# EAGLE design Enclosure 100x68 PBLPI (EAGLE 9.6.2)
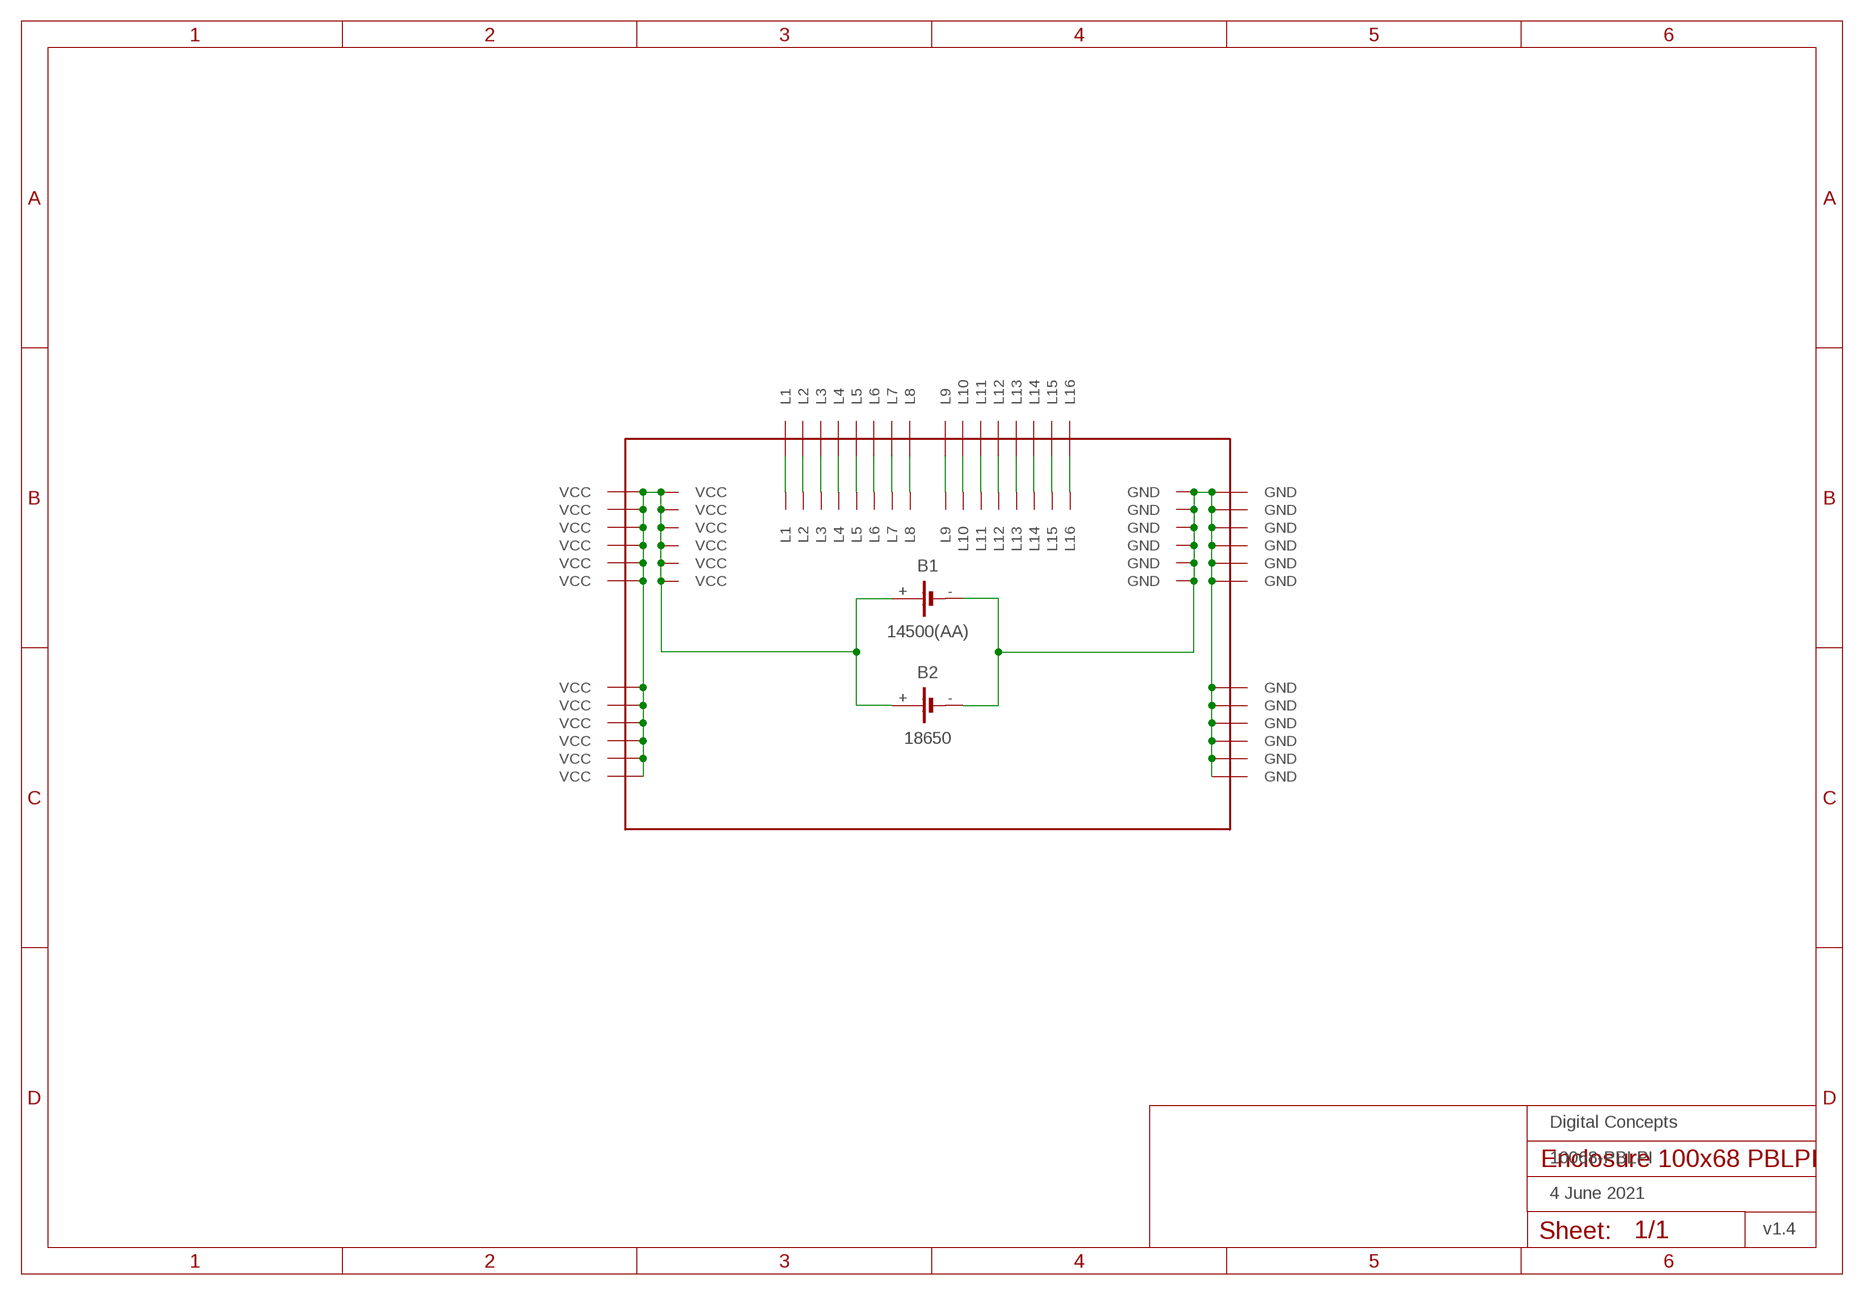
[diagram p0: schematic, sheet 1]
FRAME1 (FRAME-A4L-LOC): DATE: 4 June 2021; OWNER: Digital Concepts; TITLE: 10068-PBLPI; VERSION: v1.4

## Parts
B1  14500(AA)  BATTERY-HOLDER-14500(AA)  [BATTERY-14500]
B2  18650  BATTERY-HOLDER-18650  [BATTERY-18650]
P1  PROTO-34X22-BAT-PI  [PROTO-34X22-BAT-PI]

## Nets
GND: B1.- B2.- P1.P33-13(GND) P1.P33-14(GND) P1.P33-15(GND) P1.P33-16(GND) P1.P33-17(GND) P1.P33-18(GND) P1.P34-05(GND) P1.P34-06(GND) P1.P34-07(GND) P1.P34-08(GND) P1.P34-09(GND) P1.P34-10(GND) P1.P34-13(GND) P1.P34-14(GND) P1.P34-15(GND) P1.P34-16(GND) P1.P34-17(GND) P1.P34-18(GND)
N$1: P1.P10-21(L1) P1.P10-22(L1)
N$2: P1.P11-21(L2) P1.P11-22(L2)
N$3: P1.P12-21(L3) P1.P12-22(L3)
N$4: P1.P13-21(L4) P1.P13-22(L4)
N$5: P1.P14-21(L5) P1.P14-22(L5)
N$6: P1.P15-21(L6) P1.P15-22(L6)
N$7: P1.P16-21(L7) P1.P16-22(L7)
N$8: P1.P17-21(L8) P1.P17-22(L8)
N$9: P1.P18-21(L9) P1.P18-22(L9)
N$10: P1.P19-21(L10) P1.P19-22(L10)
N$11: P1.P20-21(L11) P1.P20-22(L11)
N$12: P1.P21-21(L12) P1.P21-22(L12)
N$13: P1.P22-21(L13) P1.P22-22(L13)
N$14: P1.P23-21(L14) P1.P23-22(L14)
N$15: P1.P24-21(L15) P1.P24-22(L15)
N$16: P1.P25-21(L16) P1.P25-22(L16)
VCC: B1.+ B2.+ P1.P01-05(VCC) P1.P01-06(VCC) P1.P01-07(VCC) P1.P01-08(VCC) P1.P01-09(VCC) P1.P01-10(VCC) P1.P01-13(VCC) P1.P01-14(VCC) P1.P01-15(VCC) P1.P01-16(VCC) P1.P01-17(VCC) P1.P01-18(VCC) P1.P02-13(VCC) P1.P02-14(VCC) P1.P02-15(VCC) P1.P02-16(VCC) P1.P02-17(VCC) P1.P02-18(VCC)

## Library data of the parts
B1 = digitalconcepts:BATTERY-HOLDER-14500(AA): 14500 (AA) battery holder
B2 = digitalconcepts:BATTERY-HOLDER-18650: 18650 Battery Holder
P1 = digitalconcepts:PROTO-34X22-BAT-PI: 34 x 22 Prototyping board, with battery connection (GND + Vcc plane), coupled side connection and Raspberry Pi Zero standoff mounting points, to fit a 100 x 68 enclosure

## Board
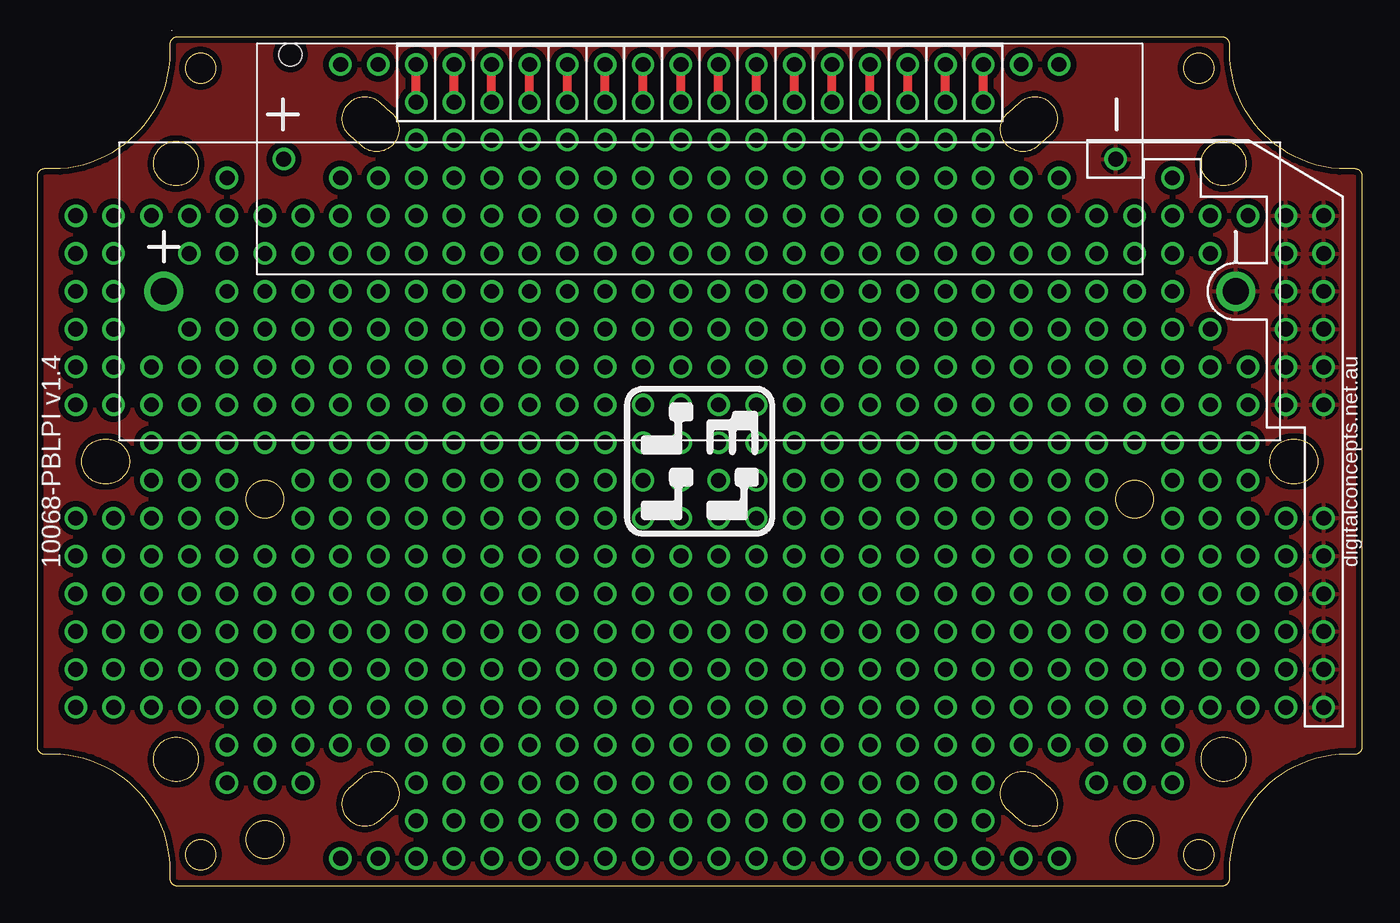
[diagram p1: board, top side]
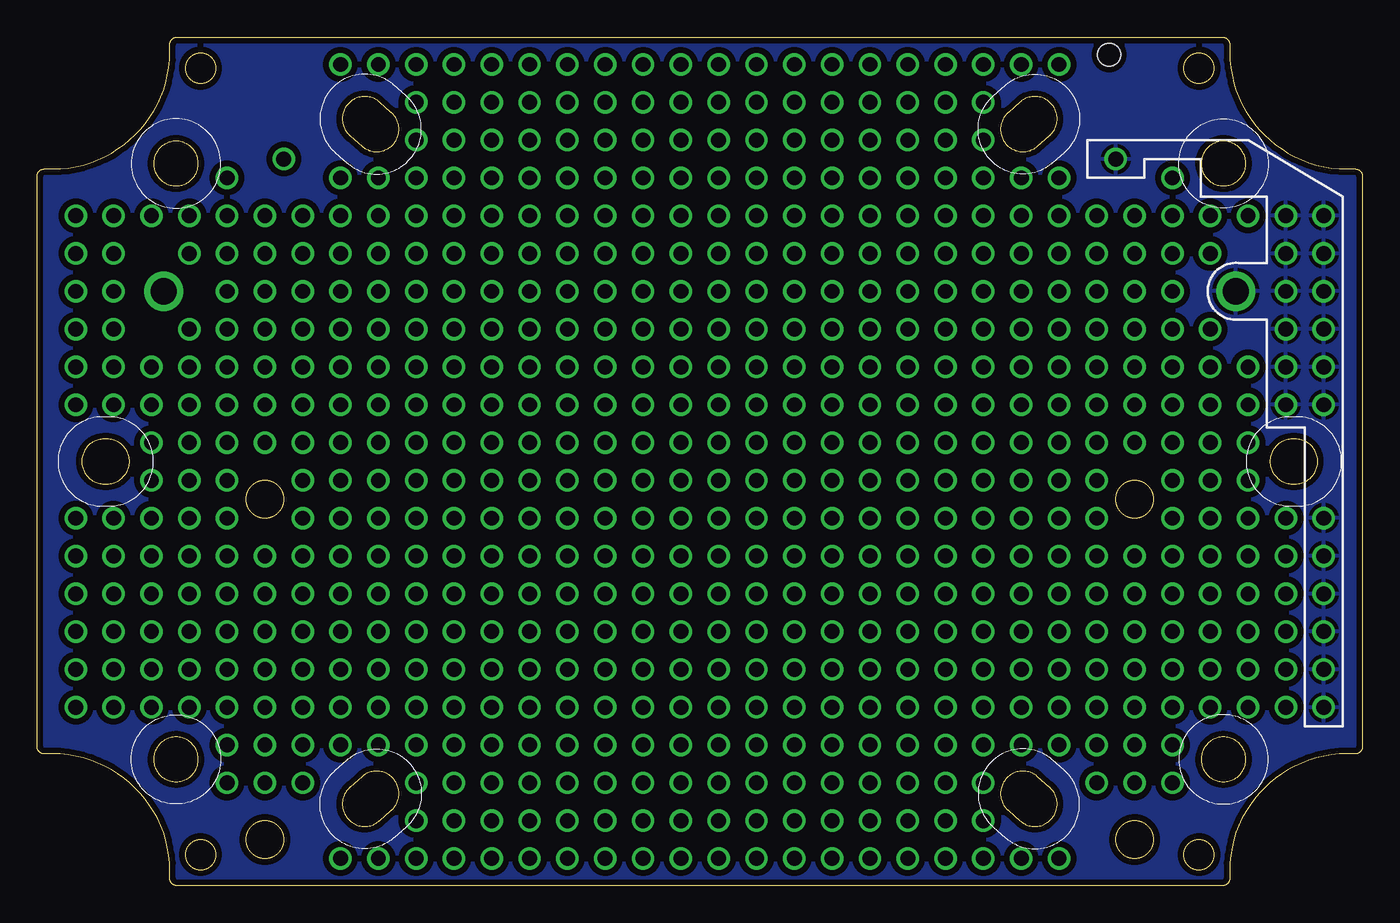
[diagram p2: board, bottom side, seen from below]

Size 89 x 57 mm. Coordinates in mm from the lower left corner, seen from the top.
Outline: 1238 segments
Outline: circle at 15.29,25.96 radius 1.27
Outline: circle at 15.29,3.1 radius 1.27
Outline: circle at 73.71,3.1 radius 1.27
Outline: circle at 73.71,25.96 radius 1.27
Outline: circle at 10.97,54.92 radius 1.02
Outline: circle at 10.97,2.08 radius 1.02
Outline: circle at 78.03,2.08 radius 1.02
Outline: circle at 78.03,54.92 radius 1.02
Copper layers (1*16): Top 0.035mm / dielectric 1.5mm / Bottom 0.035mm
Design rules "default *": minimum track width 6mil, minimum drill 0.35mm, track to track 6mil, track to pad 6mil, pad to pad 6mil, via to via 6mil, smd to smd 6mil, copper to edge 6mil, drill to drill 6mil, minimum pad ring 10mil, minimum via ring 8mil, stop-mask expansion 4mil, vias tented up to drill 0mil, thermal gap 10mil

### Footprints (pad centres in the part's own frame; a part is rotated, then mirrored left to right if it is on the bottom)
BATTERY-14500 = drill 1: + -27.94,0; - 27.94,0 | hole 1.524: -27.5,7
BATTERY-18650 = drill 1.75: + -36,0; - 36,0
PROTO-34X22-BAT-PI = drill 1: P01-05 -39.37,-13.97; P01-06 -39.37,-11.43; P01-07 -39.37,-8.89; P01-08 -39.37,-6.35; P01-09 -39.37,-3.81; P01-10 -39.37,-1.27; P01-13 -39.37,6.35; P01-14 -39.37,8.89; P01-15 -39.37,11.43; P01-16 -39.37,13.97; P01-17 -39.37,16.51; P01-18 -39.37,19.05; P02-05 -36.83,-13.97; P02-06 -36.83,-11.43; P02-07 -36.83,-8.89; P02-08 -36.83,-6.35; P02-09 -36.83,-3.81; P02-10 -36.83,-1.27; P02-13 -36.83,6.35; P02-14 -36.83,8.89; P02-15 -36.83,11.43; P02-16 -36.83,13.97; P02-17 -36.83,16.51; P02-18 -36.83,19.05; P03-05 -34.29,-13.97; P03-06 -34.29,-11.43; P03-07 -34.29,-8.89; P03-08 -34.29,-6.35; P03-09 -34.29,-3.81; P03-10 -34.29,-1.27; P03-11 -34.29,1.27; P03-12 -34.29,3.81; P03-13 -34.29,6.35; P03-14 -34.29,8.89; P03-18 -34.29,19.05; P04-05 -31.75,-13.97; P04-06 -31.75,-11.43; P04-07 -31.75,-8.89; P04-08 -31.75,-6.35; P04-09 -31.75,-3.81; P04-10 -31.75,-1.27; P04-11 -31.75,1.27; P04-12 -31.75,3.81; P04-13 -31.75,6.35; P04-14 -31.75,8.89; P04-15 -31.75,11.43; P04-17 -31.75,16.51; P04-18 -31.75,19.05; P05-03 -29.21,-19.05; P05-04 -29.21,-16.51; P05-05 -29.21,-13.97; P05-06 -29.21,-11.43; P05-07 -29.21,-8.89; P05-08 -29.21,-6.35; P05-09 -29.21,-3.81; P05-10 -29.21,-1.27; P05-11 -29.21,1.27; P05-12 -29.21,3.81; P05-13 -29.21,6.35; P05-14 -29.21,8.89; P05-15 -29.21,11.43; P05-16 -29.21,13.97; P05-17 -29.21,16.51; P05-18 -29.21,19.05; P05-19 -29.21,21.59; P06-03 -26.67,-19.05; P06-04 -26.67,-16.51; P06-05 -26.67,-13.97; P06-06 -26.67,-11.43; P06-07 -26.67,-8.89; P06-08 -26.67,-6.35; P06-09 -26.67,-3.81; P06-12 -26.67,3.81; P06-13 -26.67,6.35; P06-14 -26.67,8.89; P06-15 -26.67,11.43; P06-16 -26.67,13.97; P06-17 -26.67,16.51; P06-18 -26.67,19.05; P07-03 -24.13,-19.05; P07-04 -24.13,-16.51; P07-05 -24.13,-13.97; P07-06 -24.13,-11.43; P07-07 -24.13,-8.89; P07-08 -24.13,-6.35; P07-09 -24.13,-3.81; P07-10 -24.13,-1.27; P07-11 -24.13,1.27; P07-12 -24.13,3.81; P07-13 -24.13,6.35; P07-14 -24.13,8.89; P07-15 -24.13,11.43; P07-16 -24.13,13.97; P07-17 -24.13,16.51; P07-18 -24.13,19.05; P08-01 -21.59,-24.13; P08-04 -21.59,-16.51; P08-05 -21.59,-13.97; P08-06 -21.59,-11.43; P08-07 -21.59,-8.89; P08-08 -21.59,-6.35; P08-09 -21.59,-3.81; P08-10 -21.59,-1.27; P08-11 -21.59,1.27; P08-12 -21.59,3.81; P08-13 -21.59,6.35; P08-14 -21.59,8.89; P08-15 -21.59,11.43; P08-16 -21.59,13.97; P08-17 -21.59,16.51; P08-18 -21.59,19.05; P08-19 -21.59,21.59; P08-22 -21.59,29.21; P09-01 -19.05,-24.13; P09-04 -19.05,-16.51; P09-05 -19.05,-13.97; P09-06 -19.05,-11.43; P09-07 -19.05,-8.89; P09-08 -19.05,-6.35; P09-09 -19.05,-3.81; P09-10 -19.05,-1.27; P09-11 -19.05,1.27; P09-12 -19.05,3.81; P09-13 -19.05,6.35; P09-14 -19.05,8.89; P09-15 -19.05,11.43; P09-16 -19.05,13.97; P09-17 -19.05,16.51; P09-18 -19.05,19.05; P09-19 -19.05,21.59; P09-22 -19.05,29.21; P10-01 -16.51,-24.13; P10-02 -16.51,-21.59; P10-03 -16.51,-19.05; P10-04 -16.51,-16.51; P10-05 -16.51,-13.97; P10-06 -16.51,-11.43; P10-07 -16.51,-8.89; P10-08 -16.51,-6.35; P10-09 -16.51,-3.81; P10-10 -16.51,-1.27; P10-11 -16.51,1.27; P10-12 -16.51,3.81; P10-13 -16.51,6.35; P10-14 -16.51,8.89; P10-15 -16.51,11.43; P10-16 -16.51,13.97; P10-17 -16.51,16.51; P10-18 -16.51,19.05; P10-19 -16.51,21.59; P10-20 -16.51,24.13; P10-21 -16.51,26.67; P10-22 -16.51,29.21; P11-01 -13.97,-24.13; P11-02 -13.97,-21.59; P11-03 -13.97,-19.05; P11-04 -13.97,-16.51; P11-05 -13.97,-13.97; P11-06 -13.97,-11.43; P11-07 -13.97,-8.89; P11-08 -13.97,-6.35; P11-09 -13.97,-3.81; P11-10 -13.97,-1.27; P11-11 -13.97,1.27; P11-12 -13.97,3.81; P11-13 -13.97,6.35; P11-14 -13.97,8.89; P11-15 -13.97,11.43; P11-16 -13.97,13.97; P11-17 -13.97,16.51; P11-18 -13.97,19.05; P11-19 -13.97,21.59; P11-20 -13.97,24.13; P11-21 -13.97,26.67; P11-22 -13.97,29.21; P12-01 -11.43,-24.13; P12-02 -11.43,-21.59; P12-03 -11.43,-19.05; P12-04 -11.43,-16.51; P12-05 -11.43,-13.97; P12-06 -11.43,-11.43; P12-07 -11.43,-8.89; P12-08 -11.43,-6.35; P12-09 -11.43,-3.81; P12-10 -11.43,-1.27; P12-11 -11.43,1.27; P12-12 -11.43,3.81; P12-13 -11.43,6.35; P12-14 -11.43,8.89; P12-15 -11.43,11.43; P12-16 -11.43,13.97; P12-17 -11.43,16.51; P12-18 -11.43,19.05; P12-19 -11.43,21.59; P12-20 -11.43,24.13; P12-21 -11.43,26.67; P12-22 -11.43,29.21; P13-01 -8.89,-24.13; P13-02 -8.89,-21.59; P13-03 -8.89,-19.05; P13-04 -8.89,-16.51; P13-05 -8.89,-13.97; P13-06 -8.89,-11.43; P13-07 -8.89,-8.89; P13-08 -8.89,-6.35; P13-09 -8.89,-3.81; P13-10 -8.89,-1.27; P13-11 -8.89,1.27; P13-12 -8.89,3.81; P13-13 -8.89,6.35; P13-14 -8.89,8.89; P13-15 -8.89,11.43; P13-16 -8.89,13.97; P13-17 -8.89,16.51; P13-18 -8.89,19.05; P13-19 -8.89,21.59; P13-20 -8.89,24.13; P13-21 -8.89,26.67; P13-22 -8.89,29.21; P14-01 -6.35,-24.13; P14-02 -6.35,-21.59; P14-03 -6.35,-19.05; P14-04 -6.35,-16.51; P14-05 -6.35,-13.97; P14-06 -6.35,-11.43; P14-07 -6.35,-8.89; P14-08 -6.35,-6.35; P14-09 -6.35,-3.81; P14-10 -6.35,-1.27; P14-11 -6.35,1.27; P14-12 -6.35,3.81; P14-13 -6.35,6.35; P14-14 -6.35,8.89; P14-15 -6.35,11.43; P14-16 -6.35,13.97; P14-17 -6.35,16.51; P14-18 -6.35,19.05; P14-19 -6.35,21.59; P14-20 -6.35,24.13; P14-21 -6.35,26.67; P14-22 -6.35,29.21; P15-01 -3.81,-24.13; P15-02 -3.81,-21.59; P15-03 -3.81,-19.05; P15-04 -3.81,-16.51; P15-05 -3.81,-13.97; P15-06 -3.81,-11.43; P15-07 -3.81,-8.89; P15-08 -3.81,-6.35; P15-09 -3.81,-3.81; P15-10 -3.81,-1.27; P15-11 -3.81,1.27; P15-12 -3.81,3.81; P15-13 -3.81,6.35; P15-14 -3.81,8.89; P15-15 -3.81,11.43; P15-16 -3.81,13.97; P15-17 -3.81,16.51; P15-18 -3.81,19.05; P15-19 -3.81,21.59; P15-20 -3.81,24.13; P15-21 -3.81,26.67; P15-22 -3.81,29.21; P16-01 -1.27,-24.13; P16-02 -1.27,-21.59; P16-03 -1.27,-19.05; P16-04 -1.27,-16.51; P16-05 -1.27,-13.97; P16-06 -1.27,-11.43; P16-07 -1.27,-8.89; P16-08 -1.27,-6.35; P16-09 -1.27,-3.81; P16-10 -1.27,-1.27; P16-11 -1.27,1.27; P16-12 -1.27,3.81; P16-13 -1.27,6.35; P16-14 -1.27,8.89; P16-15 -1.27,11.43; P16-16 -1.27,13.97; P16-17 -1.27,16.51; P16-18 -1.27,19.05; P16-19 -1.27,21.59; P16-20 -1.27,24.13; P16-21 -1.27,26.67; P16-22 -1.27,29.21; P17-01 1.27,-24.13; P17-02 1.27,-21.59; P17-03 1.27,-19.05; P17-04 1.27,-16.51; P17-05 1.27,-13.97; P17-06 1.27,-11.43; P17-07 1.27,-8.89; P17-08 1.27,-6.35; P17-09 1.27,-3.81; P17-10 1.27,-1.27; P17-11 1.27,1.27; P17-12 1.27,3.81; P17-13 1.27,6.35; P17-14 1.27,8.89; P17-15 1.27,11.43; P17-16 1.27,13.97; P17-17 1.27,16.51; P17-18 1.27,19.05; P17-19 1.27,21.59; P17-20 1.27,24.13; P17-21 1.27,26.67; P17-22 1.27,29.21; P18-01 3.81,-24.13; P18-02 3.81,-21.59; P18-03 3.81,-19.05; P18-04 3.81,-16.51; P18-05 3.81,-13.97; P18-06 3.81,-11.43; P18-07 3.81,-8.89; P18-08 3.81,-6.35; P18-09 3.81,-3.81; P18-10 3.81,-1.27; P18-11 3.81,1.27; P18-12 3.81,3.81; P18-13 3.81,6.35; P18-14 3.81,8.89; P18-15 3.81,11.43; P18-16 3.81,13.97; P18-17 3.81,16.51; P18-18 3.81,19.05; P18-19 3.81,21.59; P18-20 3.81,24.13; P18-21 3.81,26.67; P18-22 3.81,29.21; P19-01 6.35,-24.13; P19-02 6.35,-21.59; P19-03 6.35,-19.05; P19-04 6.35,-16.51; P19-05 6.35,-13.97; P19-06 6.35,-11.43; P19-07 6.35,-8.89; P19-08 6.35,-6.35; P19-09 6.35,-3.81; P19-10 6.35,-1.27; P19-11 6.35,1.27; P19-12 6.35,3.81; P19-13 6.35,6.35; P19-14 6.35,8.89; P19-15 6.35,11.43; P19-16 6.35,13.97; P19-17 6.35,16.51; P19-18 6.35,19.05; P19-19 6.35,21.59; P19-20 6.35,24.13; P19-21 6.35,26.67; P19-22 6.35,29.21; P20-01 8.89,-24.13; P20-02 8.89,-21.59; P20-03 8.89,-19.05; P20-04 8.89,-16.51; P20-05 8.89,-13.97; P20-06 8.89,-11.43; P20-07 8.89,-8.89; P20-08 8.89,-6.35; P20-09 8.89,-3.81; P20-10 8.89,-1.27; P20-11 8.89,1.27; P20-12 8.89,3.81; P20-13 8.89,6.35; P20-14 8.89,8.89; P20-15 8.89,11.43; P20-16 8.89,13.97; P20-17 8.89,16.51; P20-18 8.89,19.05; P20-19 8.89,21.59; P20-20 8.89,24.13; P20-21 8.89,26.67; P20-22 8.89,29.21; P21-01 11.43,-24.13; P21-02 11.43,-21.59; P21-03 11.43,-19.05; P21-04 11.43,-16.51; P21-05 11.43,-13.97; P21-06 11.43,-11.43; P21-07 11.43,-8.89; P21-08 11.43,-6.35; P21-09 11.43,-3.81; P21-10 11.43,-1.27; P21-11 11.43,1.27; P21-12 11.43,3.81; P21-13 11.43,6.35; P21-14 11.43,8.89; P21-15 11.43,11.43; P21-16 11.43,13.97; P21-17 11.43,16.51; P21-18 11.43,19.05; P21-19 11.43,21.59; P21-20 11.43,24.13; P21-21 11.43,26.67; P21-22 11.43,29.21; P22-01 13.97,-24.13; P22-02 13.97,-21.59; P22-03 13.97,-19.05; P22-04 13.97,-16.51; P22-05 13.97,-13.97; P22-06 13.97,-11.43; P22-07 13.97,-8.89; P22-08 13.97,-6.35; P22-09 13.97,-3.81; P22-10 13.97,-1.27; P22-11 13.97,1.27; P22-12 13.97,3.81; P22-13 13.97,6.35; P22-14 13.97,8.89; P22-15 13.97,11.43; P22-16 13.97,13.97; P22-17 13.97,16.51; P22-18 13.97,19.05; P22-19 13.97,21.59; P22-20 13.97,24.13; P22-21 13.97,26.67; P22-22 13.97,29.21; P23-01 16.51,-24.13; P23-02 16.51,-21.59; P23-03 16.51,-19.05; P23-04 16.51,-16.51; P23-05 16.51,-13.97; P23-06 16.51,-11.43; P23-07 16.51,-8.89; P23-08 16.51,-6.35; P23-09 16.51,-3.81; P23-10 16.51,-1.27; P23-11 16.51,1.27; P23-12 16.51,3.81; P23-13 16.51,6.35; P23-14 16.51,8.89; P23-15 16.51,11.43; P23-16 16.51,13.97; P23-17 16.51,16.51; P23-18 16.51,19.05; P23-19 16.51,21.59; P23-20 16.51,24.13; P23-21 16.51,26.67; P23-22 16.51,29.21; P24-01 19.05,-24.13; P24-02 19.05,-21.59; P24-03 19.05,-19.05; P24-04 19.05,-16.51; P24-05 19.05,-13.97; P24-06 19.05,-11.43; P24-07 19.05,-8.89; P24-08 19.05,-6.35; P24-09 19.05,-3.81; P24-10 19.05,-1.27; P24-11 19.05,1.27; P24-12 19.05,3.81; P24-13 19.05,6.35; P24-14 19.05,8.89; P24-15 19.05,11.43; P24-16 19.05,13.97; P24-17 19.05,16.51; P24-18 19.05,19.05; P24-19 19.05,21.59; P24-20 19.05,24.13; P24-21 19.05,26.67; P24-22 19.05,29.21; P25-01 21.59,-24.13; P25-02 21.59,-21.59; P25-03 21.59,-19.05; P25-04 21.59,-16.51; P25-05 21.59,-13.97; P25-06 21.59,-11.43; P25-07 21.59,-8.89; P25-08 21.59,-6.35; P25-09 21.59,-3.81; P25-10 21.59,-1.27; P25-11 21.59,1.27; P25-12 21.59,3.81; P25-13 21.59,6.35; P25-14 21.59,8.89; P25-15 21.59,11.43; P25-16 21.59,13.97; P25-17 21.59,16.51; P25-18 21.59,19.05; P25-19 21.59,21.59; P25-20 21.59,24.13; P25-21 21.59,26.67; P25-22 21.59,29.21; P26-01 24.13,-24.13; P26-04 24.13,-16.51; P26-05 24.13,-13.97; P26-06 24.13,-11.43; P26-07 24.13,-8.89; P26-08 24.13,-6.35; P26-09 24.13,-3.81; P26-10 24.13,-1.27; P26-11 24.13,1.27; P26-12 24.13,3.81; P26-13 24.13,6.35; P26-14 24.13,8.89; P26-15 24.13,11.43; P26-16 24.13,13.97; P26-17 24.13,16.51; P26-18 24.13,19.05; P26-19 24.13,21.59; P26-22 24.13,29.21; P27-01 26.67,-24.13; P27-04 26.67,-16.51; P27-05 26.67,-13.97; P27-06 26.67,-11.43; P27-07 26.67,-8.89; P27-08 26.67,-6.35; P27-09 26.67,-3.81; P27-10 26.67,-1.27; P27-11 26.67,1.27; P27-12 26.67,3.81; P27-13 26.67,6.35; P27-14 26.67,8.89; P27-15 26.67,11.43; P27-16 26.67,13.97; P27-17 26.67,16.51; P27-18 26.67,19.05; P27-19 26.67,21.59; P27-22 26.67,29.21; P28-03 29.21,-19.05; P28-04 29.21,-16.51; P28-05 29.21,-13.97; P28-06 29.21,-11.43; P28-07 29.21,-8.89; P28-08 29.21,-6.35; P28-09 29.21,-3.81; P28-10 29.21,-1.27; P28-11 29.21,1.27; P28-12 29.21,3.81; P28-13 29.21,6.35; P28-14 29.21,8.89; P28-15 29.21,11.43; P28-16 29.21,13.97; P28-17 29.21,16.51; P28-18 29.21,19.05; P29-03 31.75,-19.05; P29-04 31.75,-16.51; P29-05 31.75,-13.97; P29-06 31.75,-11.43; P29-07 31.75,-8.89; P29-08 31.75,-6.35; P29-09 31.75,-3.81; P29-12 31.75,3.81; P29-13 31.75,6.35; P29-14 31.75,8.89; P29-15 31.75,11.43; P29-16 31.75,13.97; P29-17 31.75,16.51; P29-18 31.75,19.05; P30-03 34.29,-19.05; P30-04 34.29,-16.51; P30-05 34.29,-13.97; P30-06 34.29,-11.43; P30-07 34.29,-8.89; P30-08 34.29,-6.35; P30-09 34.29,-3.81; P30-10 34.29,-1.27; P30-11 34.29,1.27; P30-12 34.29,3.81; P30-13 34.29,6.35; P30-14 34.29,8.89; P30-15 34.29,11.43; P30-16 34.29,13.97; P30-17 34.29,16.51; P30-18 34.29,19.05; P30-19 34.29,21.59; P31-05 36.83,-13.97; P31-06 36.83,-11.43; P31-07 36.83,-8.89; P31-08 36.83,-6.35; P31-09 36.83,-3.81; P31-10 36.83,-1.27; P31-11 36.83,1.27; P31-12 36.83,3.81; P31-13 36.83,6.35; P31-14 36.83,8.89; P31-15 36.83,11.43; P31-17 36.83,16.51; P31-18 36.83,19.05; P32-05 39.37,-13.97; P32-06 39.37,-11.43; P32-07 39.37,-8.89; P32-08 39.37,-6.35; P32-09 39.37,-3.81; P32-10 39.37,-1.27; P32-11 39.37,1.27; P32-12 39.37,3.81; P32-13 39.37,6.35; P32-14 39.37,8.89; P32-18 39.37,19.05; P33-05 41.91,-13.97; P33-06 41.91,-11.43; P33-07 41.91,-8.89; P33-08 41.91,-6.35; P33-09 41.91,-3.81; P33-10 41.91,-1.27; P33-13 41.91,6.35; P33-14 41.91,8.89; P33-15 41.91,11.43; P33-16 41.91,13.97; P33-17 41.91,16.51; P33-18 41.91,19.05; P34-05 44.45,-13.97; P34-06 44.45,-11.43; P34-07 44.45,-8.89; P34-08 44.45,-6.35; P34-09 44.45,-3.81; P34-10 44.45,-1.27; P34-13 44.45,6.35; P34-14 44.45,8.89; P34-15 44.45,11.43; P34-16 44.45,13.97; P34-17 44.45,16.51; P34-18 44.45,19.05

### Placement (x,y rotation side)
B1  44.5,48.82 0 top
B2  44.5,39.93 0 top
P1  41.96,25.96 0 top

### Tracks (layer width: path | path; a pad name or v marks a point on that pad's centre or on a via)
GND
  pour Top (isolate 0.406): -1.98,58.98 -1.98,-1.98 91.11,-1.98 91.11,58.98
N$1
  Top 0.61: P1.P10-21 P1.P10-22
N$2
  Top 0.61: P1.P11-21 P1.P11-22
N$3
  Top 0.61: P1.P12-21 P1.P12-22
N$4
  Top 0.61: P1.P13-21 P1.P13-22
N$5
  Top 0.61: P1.P14-21 P1.P14-22
N$6
  Top 0.61: P1.P15-21 P1.P15-22
N$7
  Top 0.61: P1.P16-21 P1.P16-22
N$8
  Top 0.61: P1.P17-21 P1.P17-22
N$9
  Top 0.61: P1.P18-21 P1.P18-22
N$10
  Top 0.61: P1.P19-21 P1.P19-22
N$11
  Top 0.61: P1.P20-21 P1.P20-22
N$12
  Top 0.61: P1.P21-21 P1.P21-22
N$13
  Top 0.61: P1.P22-21 P1.P22-22
N$14
  Top 0.61: P1.P23-21 P1.P23-22
N$15
  Top 0.61: P1.P24-21 P1.P24-22
N$16
  Top 0.61: P1.P25-21 P1.P25-22
VCC
  pour Bottom (isolate 0.406): -0.71,57.71 -0.71,-0.71 89.84,-0.71 89.84,57.71

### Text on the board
tPlace: 10068-PBLPI v1.4 | digitalconcepts.net.au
